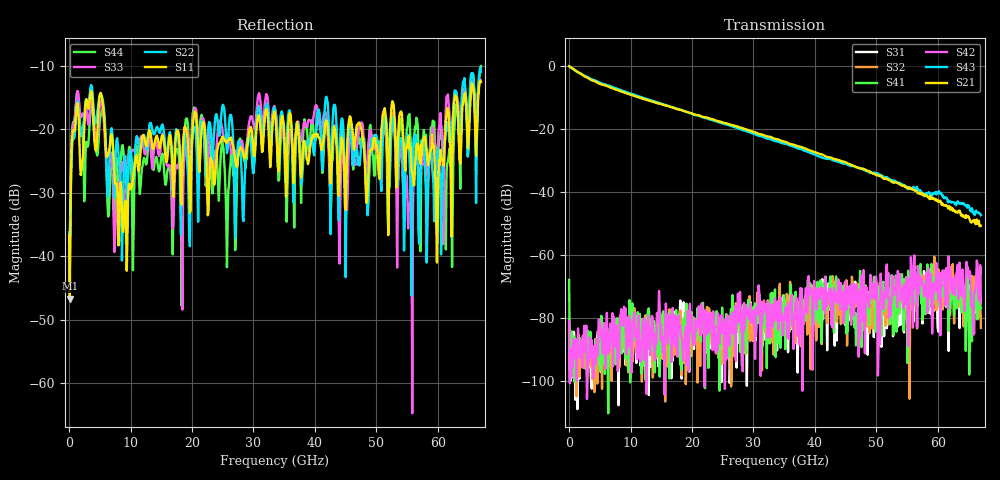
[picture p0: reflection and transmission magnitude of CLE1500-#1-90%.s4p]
!Keysight Technologies,N5247B,US50470101,A.16.20.02
!Date: Thursday, March 13, 2025 10:32:55
!Correction: S11(C  4-Port  )
!S12(C  4-Port  )
!S13(C  4-Port  )
!S14(C  4-Port  )
!S21(C  4-Port  )
!S22(C  4-Port  )
!S23(C  4-Port  )
!S24(C  4-Port  )
!S31(C  4-Port  )
!S32(C  4-Port  )
!S33(C  4-Port  )
!S34(C  4-Port  )
!S41(C  4-Port  )
!S42(C  4-Port  )
!S43(C  4-Port  )
!S44(C  4-Port  )
!S4P File: Measurements: <S11,S12,S13,S14>,
!<S21,S22,S23,S24>,
!<S31,S32,S33,S34>,
!<S41,S42,S43,S44>:
# Hz S  dB  R 50
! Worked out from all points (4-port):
!   601 points, 10 MHz to 67 GHz, reference 50 ohm
!   strongest paths, dB at 10 MHz, 16.76 GHz, 33.51 GHz, 50.25 GHz, 67 GHz:
!     S21: 0.0, -13.1, -23.0, -34.7, -50.6
!     S43: 0.0, -13.0, -23.8, -34.1, -47.3
!     S42: -80.9, -78.2, -73.6, -98.1, -75.2
!     S41: -67.8, -78.0, -70.8, -82.8, -76.7
!     S32: -80.4, -81.6, -80.6, -70.1, -83.1
!     S31: -84.3, -78.4, -88.6, -71.5, -64.0
!   lowest |S11| = -46.7 dB at 121.7 MHz (marker M1), VSWR 1.01, Z = 49.7 - j0.37 ohm
!   |S11| at or under -10 dB: start of sweep to end of sweep
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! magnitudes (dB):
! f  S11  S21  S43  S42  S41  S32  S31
! 10 MHz  -36.7  0.0  0.0  -80.9  -67.8  -80.4  -84.3
! 121.7 MHz  -46.7  -0.1  -0.2  -100.6  -91.1  -92.8  -98.7
! 3.583 GHz  -14.0  -4.4  -4.1  -92.4  -90.0  -95.4  -99.8
! 9.165 GHz  -31.3  -8.5  -8.1  -76.8  -92.7  -81.3  -94.7
! 30.94 GHz  -17.9  -21.5  -22.2  -71.6  -72.3  -79.0  -80.9
! 55.5 GHz  -22.8  -39.0  -38.5  -72.7  -73.9  -78.0  -71.5
! 67 GHz  -12.6  -50.6  -47.3  -75.2  -76.7  -83.1  -64.0
